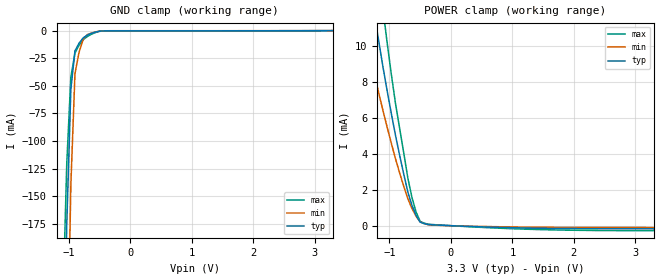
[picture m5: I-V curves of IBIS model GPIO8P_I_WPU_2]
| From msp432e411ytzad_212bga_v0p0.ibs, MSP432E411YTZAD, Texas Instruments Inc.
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|   Model Cell GPIO8P_I_WPU_2
[Model]   GPIO8P_I_WPU_2
Model_type   Input
Polarity   Non-Inverting
Vinl =  0.8
Vinh =  2
C_comp   5.378567p   4.597605p   6.118031p
[Model Spec]
Vinl   0.8   0.8   0.8
Vinh   2   2   2
[Temperature Range]   25   125   -40
[Voltage Range]   3.3   2.97   3.63
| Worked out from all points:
|   GND clamp passes 1 mA (typ) near -0.54 V on its own axis
|   POWER clamp passes 1 mA (typ) near -0.62 V on its own axis
| Nom Voltages:
|   VBAT=3.3, VDDC=1.2, VDD=3.3, GND=0
| Min Voltages:
|   VBAT=2.97, VDDC=1.08, VDD=2.97, GND=0
| Max Voltages:
|   VBAT=3.63, VDDC=1.32, VDD=3.63, GND=0
[POWER_clamp]
|   voltage   I(typ)   I(min)   I(max)
-3.3V     116.2mA    496.9mA    244.4mA
-1.433V   16.06mA    11.3mA     22.46mA
-1.367V   14.5mA     10.25mA    20.22mA
-1.233V   11.51mA    8.234mA    15.92mA
-1.167V   10.09mA    7.266mA    13.87mA
-1.1V     8.711mA    6.319mA    11.88mA
-1.033V   7.42mA     5.419mA    10.06mA
-900mV    4.993mA    3.699mA    6.758mA
-700mV    1.865mA    1.492mA    2.636mA
-566.7mV  567.7uA    525.4uA    760.1uA
-500mV    194.9uA    210.9uA    235.6uA
3.3V      -173.5uA   -106.4uA   -276.5uA
[GND_clamp]
|   voltage   I(typ)   I(min)   I(max)
-3.3V     -16.39A    -15.37A    -17.22A
-1.1V     -384.9mA   -635.5mA   -255.1mA
-1.033V   -175.3mA   -338.1mA   -120.1mA
-966.7mV  -53.11mA   -139.3mA   -41.82mA
-900mV    -18.35mA   -38.91mA   -20.37mA
-833.3mV  -11.37mA   -19.64mA   -13.21mA
-766.7mV  -6.606mA   -7.888mA   -8.217mA
-700mV    -4.057mA   -3.651mA   -5.393mA
-500mV    -490uA     -474.1uA   -637.3uA
-366.7mV  -189.3uA   -130.6uA   -292.3uA
3.3V      362.4pA    36.7uA     -64.12uA
